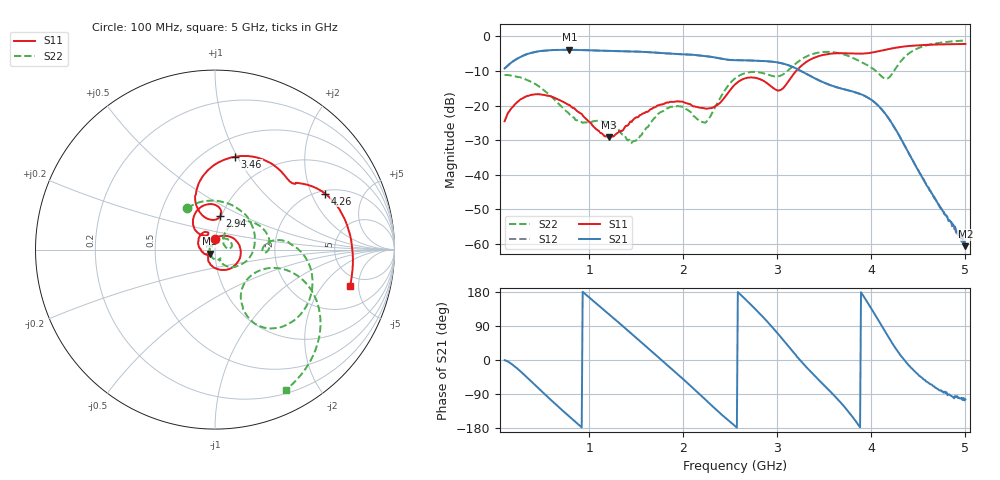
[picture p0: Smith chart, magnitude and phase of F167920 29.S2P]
!  2-Port S-parameters saved by WinCal
! VAR MeasName=S-Parameters (CALIBRATED_DATA) read from VNA (N5242A)
! VAR MeasDate=2016-11-22 9:56:35
! VAR NAME=F167920 29
! VAR FILENAME=F167920 29.S2P
! VAR DATE=2016-11-22 9:56:36
! VAR PHYS_PORTS=1,2
# Hz S DB R 50
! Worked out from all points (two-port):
!   491 points, 100 MHz to 5 GHz, reference 50 ohm
!   highest |S21| = -3.85 dB at 790 MHz (marker M1); lowest = -60.6 dB at 5 GHz (marker M2)
!   |S21| within 3 dB of the highest: 207.2 MHz to 2.553 GHz (2.345 GHz wide, 170 % of centre)
!   lowest |S11| = -29.2 dB at 1.21 GHz (marker M3), VSWR 1.07, Z = 47.3 - j2.09 ohm
!   |S11| at or under -10 dB: start of sweep to 3.199 GHz
!   |S22| runs from -30.8 to -1.2 dB; largest |S21 - S12| = 0.0011
!   S11 on the Smith chart (normalised r, x): 100 MHz: 1.00, +0.12; 2.94 GHz: 0.99, +0.38; 3.46 GHz: 0.68, +0.98; 4.26 GHz: 2.13, +2.53; 5 GHz: 3.88, -3.96
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1e8  -24.51 88.1  -9.23 -0.5  -9.23 -0.5  -11.15 123.7
3e8  -17.75 20.1  -5.51 -37.0  -5.51 -37.1  -12.19 33.3
5e8  -16.86 -29.9  -4.16 -84.1  -4.16 -84.1  -15.21 -26.4
7.9e8  -19.83 -92.8  -3.85 -149.5  -3.85 -149.5  -22.51 -65.7
9.2e8  -22.38 -118.3  -3.91 -177.7  -3.91 -177.7  -24.79 -61.7
1.21e9  -29.17 -140.7  -4.18 120.5  -4.18 120.5  -24.90 -84.4
1.47e9  -23.99 -157.7  -4.38 65.2  -4.38 65.2  -30.22 163.9
1.74e9  -19.88 157.4  -4.73 6.3  -4.73 6.2  -22.25 56.6
1.96e9  -18.80 124.7  -5.11 -41.8  -5.11 -41.8  -20.20 16.7
2.14e9  -20.38 112.5  -5.41 -82.6  -5.41 -82.7  -23.69 7.8
2.25e9  -20.87 117.6  -5.71 -108.0  -5.72 -108.1  -24.50 38.9
2.55e9  -13.89 127.5  -6.85 -174.1  -6.85 -174.2  -12.14 39.5
2.73e9  -11.85 97.7  -6.95 143.4  -6.95 143.4  -10.26 11.3
2.94e9  -14.55 81.2  -7.27 88.3  -7.28 88.3  -11.35 -3.2
3.15e9  -11.72 112.9  -8.65 26.8  -8.65 26.7  -8.93 8.6
3.37e9  -6.41 89.2  -11.68 -34.8  -11.70 -34.9  -5.11 -13.7
3.46e9  -5.52 77.8  -12.91 -57.5  -12.93 -57.5  -4.58 -25.1
3.76e9  -4.90 48.9  -15.62 -137.4  -15.63 -137.4  -5.68 -57.1
4.19e9  -3.60 31.2  -23.89 56.9  -23.94 57.2  -11.81 -30.5
4.26e9  -3.25 27.0  -26.94 30.1  -26.97 30.3  -9.19 -17.1
4.53e9  -2.50 9.8  -40.18 -45.3  -40.25 -45.1  -3.05 -33.4
5e9  -2.17 -14.9  -60.61 -103.9  -59.84 -106.9  -1.15 -63.2
